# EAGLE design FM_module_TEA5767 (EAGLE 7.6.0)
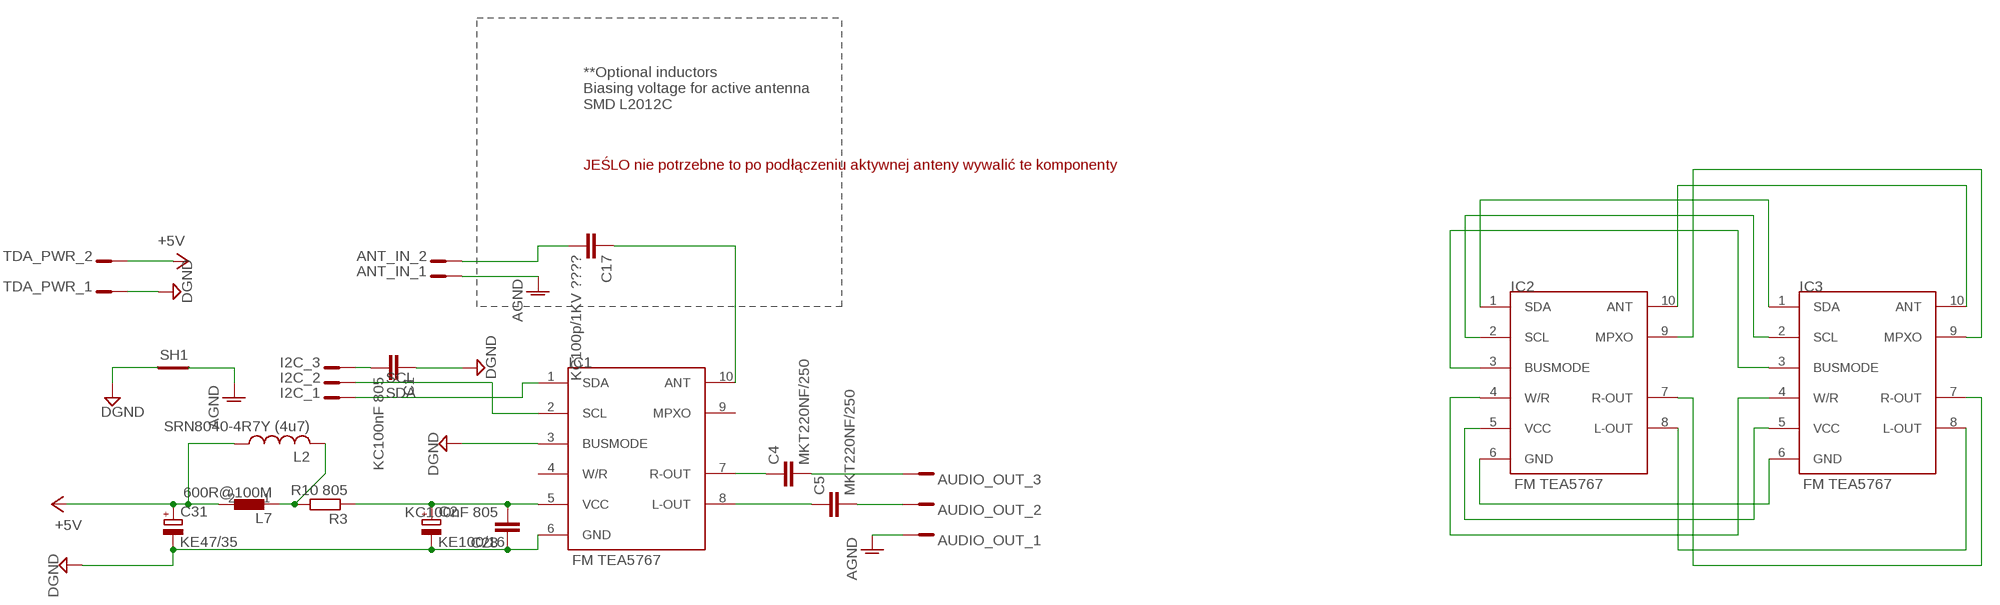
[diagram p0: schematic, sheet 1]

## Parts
ANT_IN  JST_2_PIN_B2B-PH-KS  [B2B-PH-KS]
AUDIO_OUT  JST_3_PIN_B3B-PH-KS  [B3B-PH-KS]
C1  KC100nF 805  C-EUC0805  [C0805]
C2  KE100/16  CPOL-EUTT2D6  [TT2D6]
C4  MKT220NF/250  C-EU050-050X075  [C050-050X075]
C5  MKT220NF/250  C-EU050-050X075  [C050-050X075]
C17  KC100p/1KV ????  C-EU050-025X075  [C050-025X075]
C28  KC100nF 805  C-EUC0805  [C0805]
C31  KE47/35  CPOL-EUTT2D6  [TT2D6]
I2C  JST_3_PIN_B3B-PH-KS  [B3B-PH-KS]
IC1  FM TEA5767  TEA5767_MODULE_2.54MM  [PROTOTYPE]
IC2  FM TEA5767  TEA5767_MODULE_2.54MM  [PROTOTYPE]
IC3  FM TEA5767  TEA5767_MODULE_SMD  [SMD]
L2  SRN8040-4R7Y (4u7)  L-US0204/5  [0204/5]
L7  600R@100M  FERRITR0805  [R0805]
R3  R10 805  R-EU_R0805  [R0805]
SH1  SHORT-HT5  [SHORT_TOP-50]
TDA_PWR  JST_2_PIN_B2B-XH-A  [B2B-XH-A]

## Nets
+5V: C31.+ L2.1 L7.2 TDA_PWR.P$2
AGND: ANT_IN.P$1 AUDIO_OUT.P$1 SH1.2
DGND: C1.1 C2.- C28.1 C31.- IC1.3(BUSMODE) IC1.6(GND) SH1.1 TDA_PWR.P$1
N$1: ANT_IN.P$2 C17.2
N$2: IC2.1(SDA) IC3.1(SDA)
N$4: C2.+ C28.2 IC1.5(VCC) R3.1
N$6: C17.1 IC1.10(ANT)
N$7: IC2.2(SCL) IC3.2(SCL)
N$8: C4.1 IC1.7(R-OUT)
N$9: C5.1 IC1.8(L-OUT)
N$10: IC2.3(BUSMODE) IC3.3(BUSMODE)
N$11: IC2.10(ANT) IC3.10(ANT)
N$12: IC2.9(MPXO) IC3.9(MPXO)
N$13: IC2.6(GND) IC3.6(GND)
N$14: IC2.5(VCC) IC3.5(VCC)
N$15: IC2.4(W/R) IC3.4(W/R)
N$16: L2.2 L7.1 R3.2
N$17: IC2.8(L-OUT) IC3.8(L-OUT)
N$18: IC2.7(R-OUT) IC3.7(R-OUT)
N$28: AUDIO_OUT.P$3 C4.2
N$29: AUDIO_OUT.P$2 C5.2
N$30: C1.2 I2C.P$3
SCL: I2C.P$2 IC1.2(SCL)
SDA: I2C.P$1 IC1.1(SDA)
Unconnected: IC1.4(W/R) IC1.9(MPXO)

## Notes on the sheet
- **Optional inductors
  Biasing voltage for active antenna
  SMD L2012C
- JEŚLO nie potrzebne to po podłączeniu aktywnej anteny wywalić te komponenty

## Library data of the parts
ANT_IN TDA_PWR = conn-JST:JST_2_PIN_
AUDIO_OUT I2C = conn-JST:JST_3_PIN_
C1 C4 C5 C17 C28 = rcl:C-EU: CAPACITOR, European symbol
C2 C31 = rcl:CPOL-EU: POLARIZED CAPACITOR, European symbol
IC1-IC3 = TEA5767_module:TEA5767_MODULE_
L2 = rcl:L-US: INDUCTOR, American symbol
L7 = ferrit_bear:FERRIT
R3 = rcl:R-EU_: RESISTOR, European symbol
SH1 = shorts-old:SHORT-H: Short between two nets; BOM: no

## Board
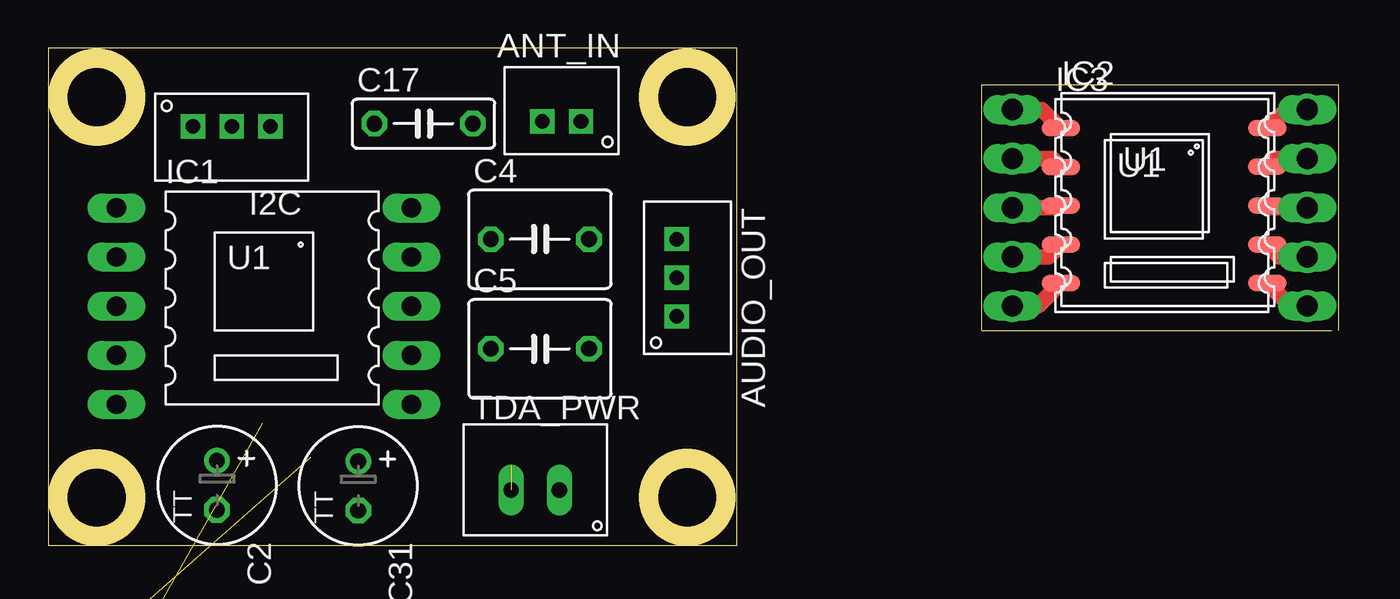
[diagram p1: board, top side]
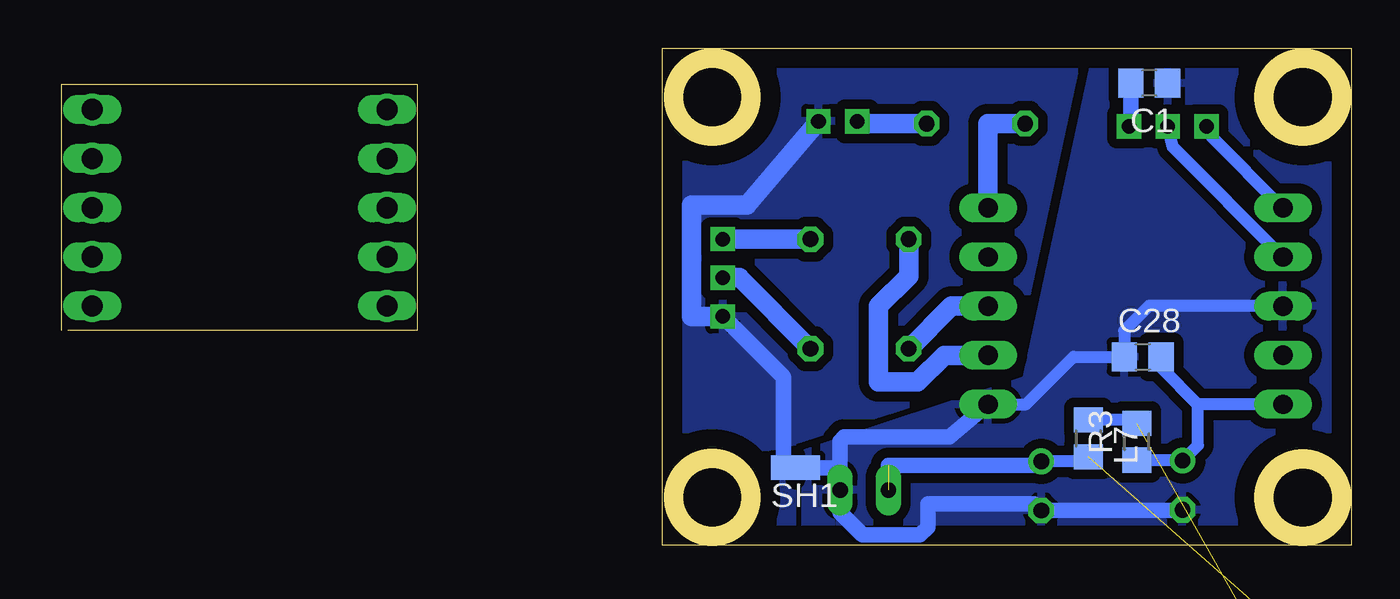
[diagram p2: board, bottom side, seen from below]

Size 66.65 x 25.7 mm. Coordinates in mm from the lower left corner, seen from the top.
Outline: 66.65,11.11 66.65,23.82 48.24,23.82 48.24,11.11 66.33,11.11
Outline: 0,0 35.58,0 35.58,25.7 0,25.7 0,0
Outline: circle at 33.01,23.18 radius 2
Outline: circle at 33.02,2.49 radius 2
Outline: circle at 2.49,23.17 radius 2
Outline: circle at 2.5,2.47 radius 2
Copper layers (1*16): Top 0.035mm / dielectric 1.5mm / Bottom 0.035mm
Design rules "default": minimum track width 10mil, minimum drill 24mil, track to track 8mil, track to pad 8mil, pad to pad 8mil, via to via 8mil, smd to smd 8mil, copper to edge 40mil, drill to drill 8mil, minimum pad ring 10mil, minimum via ring 8mil, stop-mask expansion 4mil, vias tented up to drill 0mil, thermal gap 10mil

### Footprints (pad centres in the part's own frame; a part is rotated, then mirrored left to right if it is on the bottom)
B2B-PH-KS = drill 0.75 pad 1.2 square: P$1 -2,1.7; P$2 -4,1.7
B3B-PH-KS = drill 0.75 pad 1.2 square: P$1 -2,1.7; P$2 -4,1.7; P$3 -6,1.7
C0805 = smd 1.3 x 1.5: 1 -0.95,0; 2 0.95,0
TT2D6 = drill 0.813: + -1.27,0 | drill 0.813 octagon: - 1.27,0
C050-050X075 = drill 0.813 octagon: 1 -2.54,0; 2 2.54,0
C050-025X075 = drill 0.813 octagon: 1 -2.54,0; 2 2.54,0
PROTOTYPE = drill 1 pad 1.27 long: 1 -7.62,3.81; 2 -7.62,1.27; 3 -7.62,-1.27; 4 -7.62,-3.81; 5 -7.62,-6.35; 6 7.62,-6.35; 7 7.62,-3.81; 8 7.62,-1.27; 9 7.62,1.27; 10 7.62,3.81
SMD = smd 2 x 0.85: 1 -4.8,3.15; 2 -4.8,1.15; 3 -4.8,-0.85; 4 -4.8,-2.85; 5 -4.8,-4.85; 6 5.866,-4.85; 7 5.866,-2.85; 8 5.866,-0.85; 9 5.866,1.16; 10 5.866,3.15
0204/5 = drill 0.813 octagon: 1 -2.54,0; 2 2.54,0
R0805 = smd 1.3 x 1.5: 1 -0.95,0; 2 0.95,0
SHORT_TOP-50 = smd 1.27 x 1.27: 1 0.635,0; 2 -0.635,0
B2B-XH-A = drill 0.8 long: P$1 -2.45,2.35; P$2 -4.95,2.35

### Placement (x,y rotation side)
ANT_IN  29.53,20.23 0 top
AUDIO_OUT  30.77,9.84 270 top
C1  10.43,23.91 180 bottom
C2  8.71,3.11 270 top
C4  25.4,15.84 0 top
C5  25.4,10.17 0 top
C17  19.39,21.81 0 top
C28  10.77,9.75 0 bottom
C31  16.01,3.08 270 top
I2C  5.48,23.37 180 top
IC1  11.14,13.64 0 top
IC2  57.44,18.73 0 top
IC3  57.13,18.41 0 top
L2  not placed on the board
L7  13.58,5.54 270 bottom
R3  11.08,5.36 90 bottom
SH1  28.71,4.02 0 bottom
TDA_PWR  28.86,0.52 0 top

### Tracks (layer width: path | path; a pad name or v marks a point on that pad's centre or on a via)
+5V  (2 unrouted)
  Bottom 0.61: L7.2 13.82,4.35 C31.+
  Bottom 0.813: C31.+ 16.2,4.15 23.91,4.15
AGND
  Bottom 0.813: SH1.2 29.35,8.72 AUDIO_OUT.P$1
  Bottom 1.016: AUDIO_OUT.P$1 34.09,11.84 34.09,17.6 31.22,17.6 ANT_IN.P$1
  pour Bottom (isolate 0.508): 13.88,26.39 38.73,26.39 39.04,-1.44 28.88,-1.44 28.88,5.41 20.61,8.03 20.53,8.76 17.67,8.76
DGND
  Bottom 0.61: IC1.3 10.45,12.38 11.72,11.11 C28.1 14.35,9.75 16.8,7.3 IC1.6
  Bottom 0.813: C2.- 8.71,1.81 C31.- 16.36,2.15 21.88,2.15 21.88,0.95 22.28,0.55 25.25,0.55 26.41,1.71 TDA_PWR.P$1 26.41,3.49 | IC1.6 20.76,5.6 26.2,5.6 26.41,5.39 26.41,3.49 | SH1.1 26.94,4.02 arc90 26.41,3.49
  pour Bottom (isolate 0.508): -3.52,26.35 12.99,26.35 16.8,8.55 28.23,4.76 28.23,-1.59 -3.52,-1.59
N$1
  Bottom 1.016: C17.2 25.53,21.81 ANT_IN.P$2
N$2
  Top 0.813: IC2.1 51.35,22.54 IC3.1
N$4
  Bottom 0.61: IC1.5 7.91,7.3 | 7.91,7.3 9.82,9.21 C28.2 | 7.91,7.3 7.91,5.18 C2.+ 8.74,4.41 R3.1
N$5  (via drill 1.1)
  other vias: 49.82,20
N$6
  Bottom 1.016: C17.1 18.76,21.81 IC1.10
N$7
  Top 0.813: IC2.2 51.89,20 IC3.2
N$8
  Bottom 1.016: C4.1 22.86,13.94 24.42,12.38 24.42,8.45 22.41,8.45 21.02,9.83 IC1.7
N$9
  Bottom 1.016: IC1.8 20.65,12.37 C5.1
N$10
  Top 0.813: IC2.3 52.22,17.46 IC3.3
N$11
  Top 0.813: IC2.10 63.97,22.54 IC3.10
N$12
  Top 0.813: IC2.9 63.42,20 IC3.9
N$13
  Top 0.813: IC2.6 64.18,12.38 IC3.6
N$14
  Top 0.813: IC2.5 51.14,12.38 IC3.5
N$15
  Top 0.813: IC2.4 51.68,14.92 IC3.4
N$16  (1 unrouted)
  Bottom 0.61: R3.2 11.25,6.49 L7.1
N$17
  Top 0.813: IC2.8 63.1,17.46 IC3.8
N$18
  Top 0.813: IC2.7 63.64,14.92 IC3.7
N$19  (via drill 1.1)
  other vias: 49.82,22.54
N$20  (via drill 1.1)
  other vias: 49.82,17.46
N$21  (via drill 1.1)
  other vias: 49.82,14.92
N$22  (via drill 1.1)
  other vias: 49.82,12.38
N$23  (via drill 1.1)
  other vias: 65.06,22.54
N$24  (via drill 1.1)
  other vias: 65.06,20
N$25  (via drill 1.1)
  other vias: 65.06,17.46
N$26  (via drill 1.1)
  other vias: 65.06,14.92
N$27  (via drill 1.1)
  other vias: 65.06,12.38
N$28
  Bottom 1.016: C4.2 AUDIO_OUT.P$3
N$29
  Bottom 1.016: C5.2 31.61,13.84 AUDIO_OUT.P$2
N$30
  Bottom 0.813: I2C.P$3 11.38,21.56 C1.2
SCL
  Bottom 0.61: IC1.2 9.22,20.61 I2C.P$2
SDA
  Bottom 0.61: IC1.1 7.22,21.15 I2C.P$1

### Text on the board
Document: SDA / SLC / GND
